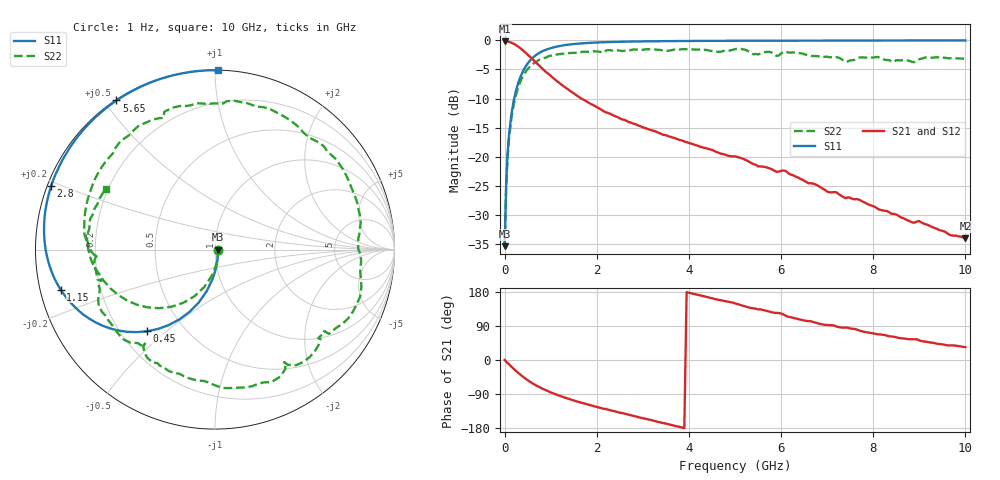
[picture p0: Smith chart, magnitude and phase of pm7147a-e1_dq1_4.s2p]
# GHz S DB R 50
! S-Parameters data
! Freq  dbS11  angS11  dbS21  angS21  dbS12  angS12  dbS22  angS22
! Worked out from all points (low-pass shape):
!   279 points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, 1 Hz to 10 GHz, reference 50 ohm
!   highest |S21| = -0.15 dB at 501.2 Hz (marker M1); lowest = -34.1 dB at 10 GHz (marker M2)
!   |S21| within 3 dB of the highest: start of sweep to 594.2 MHz
!   lowest |S11| = -35.4 dB at 199.5 Hz (marker M3), VSWR 1.03, Z = 51.7 - j3.26e-05 ohm
!   |S11| at or under -10 dB: start of sweep to 207.7 MHz
!   |S22| runs from -35.4 to -1.4 dB; largest |S21 - S12| = 0
!   S11 on the Smith chart (normalised r, x): 1 Hz: 1.03, -0.00; 450 MHz: 0.31, -0.43; 1.15 GHz: 0.06, -0.13; 2.8 GHz: 0.01, +0.19; 5.65 GHz: 0.00, +0.54; 10 GHz: 0.00, +1.02
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1e-09  -35.42 -0.0  -0.15 -0.0  -0.15 -0.0  -35.42 -0.0
1.995e-07  -35.42 -0.0  -0.15 -0.0  -0.15 -0.0  -35.42 -0.0
5.012e-07  -35.42 -0.0  -0.15 -0.0  -0.15 -0.0  -35.42 -0.0
0.03981072  -23.61 -79.0  -0.17 -4.8  -0.17 -4.8  -24.24 -79.3
0.1  -15.95 -94.2  -0.26 -12.0  -0.26 -12.0  -16.61 -97.2
0.25  -8.54 -112.2  -0.82 -29.1  -0.82 -29.1  -9.27 -120.7
0.45  -4.56 -129.7  -2.07 -48.9  -2.07 -48.9  -5.46 -144.9
0.8  -1.94 -151.3  -4.70 -74.5  -4.70 -74.5  -3.15 -176.2
1.15  -1.03 -165.5  -7.09 -92.5  -7.09 -92.5  -2.40 160.7
1.7  -0.49 179.3  -10.14 -113.7  -10.14 -113.7  -1.95 131.9
2.25  -0.28 168.1  -12.49 -131.0  -12.49 -131.0  -1.66 106.7
2.8  -0.18 158.8  -14.34 -147.6  -14.34 -147.6  -1.55 82.5
3.35  -0.13 150.7  -15.94 -164.0  -15.94 -164.0  -1.63 57.4
4.25  -0.08 139.0  -18.30 170.4  -18.30 170.4  -1.58 17.9
5.05  -0.05 129.8  -20.07 147.7  -20.07 147.7  -1.41 -17.9
5.65  -0.04 123.4  -21.79 130.7  -21.79 130.7  -2.01 -45.4
6.1  -0.03 119.0  -22.46 116.7  -22.46 116.7  -1.91 -67.0
6.7  -0.02 113.5  -24.65 100.2  -24.65 100.2  -2.68 -96.7
7.25  -0.02 108.7  -26.45 86.7  -26.45 86.7  -2.97 -122.2
8.35  -0.01 100.1  -29.60 62.5  -29.60 62.5  -3.38 -163.7
9.15  -0.00 94.5  -31.67 48.2  -31.67 48.2  -2.91 175.4
10  -0.00 89.1  -34.05 34.2  -34.05 34.2  -3.18 150.8
